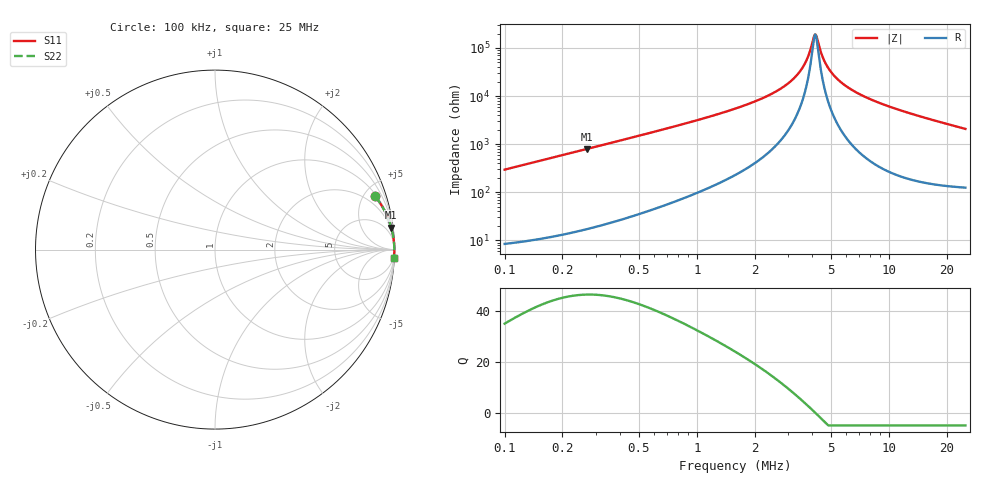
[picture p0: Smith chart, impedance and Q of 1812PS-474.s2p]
# MHz S MA R 50
!Freq  MagS11  AngS11  MagS21  AngS21  MagS12  AngS12  MagS22  AngS22
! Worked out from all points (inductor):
!   801 points, 100 kHz to 25 MHz, reference 50 ohm
!   read as one part in series: L = 470 uH near 102.8 kHz
!   highest Q = 46.5 at 268.3 kHz (marker M1), where L = 472 uH
!   self-resonance near 4.127 MHz
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0.1  0.9392 18.5  0.3177 -69.8  0.3177 -69.8  0.9392 18.5
0.2521477  0.9884 7.6  0.1322 -81.2  0.1322 -81.2  0.9884 7.6
0.2683069  0.9896 7.1  0.1244 -81.6  0.1244 -81.6  0.9896 7.1
0.6314115  0.9973 3.0  0.05225 -85.6  0.05225 -85.6  0.9973 3.0
1.581139  0.9991 1.0  0.01828 -86.6  0.01828 -86.6  0.9991 1.0
2.359504  0.9993 0.6  0.009695 -85.7  0.009695 -85.7  0.9993 0.6
2.727511  0.9994 0.4  0.007037 -84.8  0.007037 -84.8  0.9994 0.4
3.067064  0.9994 0.3  0.004999 -83.2  0.004999 -83.2  0.9994 0.3
3.354975  0.9994 0.2  0.003495 -80.8  0.003495 -80.8  0.9994 0.2
3.594708  0.9995 0.1  0.002366 -76.7  0.002366 -76.7  0.9995 0.1
3.79877  0.9995 0.1  0.001493 -69.1  0.001493 -69.1  0.9995 0.1
3.986805  0.9995 0.0  0.0007997 -48.9  0.0007997 -48.9  0.9995 0.0
4.098403  0.9995 0.0  0.0005439 -16.1  0.0005439 -16.1  0.9995 0.0
4.184147  0.9995 -0.0  0.0005534 19.8  0.0005534 19.8  0.9995 -0.0
4.242304  0.9995 -0.0  0.0006639 38.5  0.0006639 38.5  0.9995 -0.0
4.514177  0.9995 -0.1  0.001522 70.1  0.001522 70.1  0.9995 -0.1
4.737624  0.9995 -0.1  0.002285 76.9  0.002285 76.9  0.9995 -0.1
5.11131  0.9995 -0.2  0.003526 81.4  0.003526 81.4  0.9995 -0.2
5.629842  0.9995 -0.3  0.005149 83.9  0.005149 83.9  0.9995 -0.3
7.118831  0.9994 -0.5  0.00934 86.0  0.00934 86.0  0.9994 -0.5
9.983492  0.9992 -0.9  0.01636 86.6  0.01636 86.6  0.9992 -0.9
25  0.996 -2.7  0.04787 83.8  0.04787 83.8  0.996 -2.7
